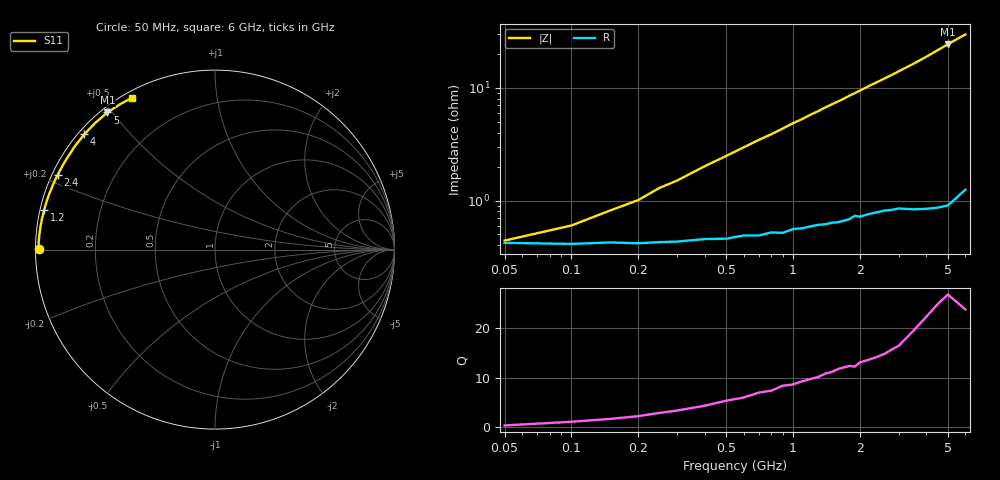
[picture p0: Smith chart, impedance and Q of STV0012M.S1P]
! SIEMENS Discrete & RF Semiconductors
! BA892
! Si PIN Diode in SCD-80
! IF = 12 mA
! S-Parameters:  September  1997
# GHz  S  MA  R  50
!  f  S11
! GHz  MAG  ANG
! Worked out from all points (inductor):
!   34 points, 50 MHz to 6 GHz, reference 50 ohm
!   read as one part to ground: L = 778 pH near 300 MHz
!   highest Q = 25.3 at 5 GHz (marker M1), where L = 774 pH
!   S11 on the Smith chart (normalised r, x): 50 MHz: 0.01, +0.00; 1.2 GHz: 0.01, +0.11; 2.4 GHz: 0.02, +0.22; 4 GHz: 0.02, +0.38; 5 GHz: 0.02, +0.49; 6 GHz: 0.02, +0.59
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0.05  0.9833 179.7
0.1  0.9837 179.0
0.15  0.9832 178.4
0.2  0.9834 177.9
0.25  0.9831 177.2
0.3  0.9829 176.7
0.4  0.982 175.5
0.7  0.9807 172.2
0.8  0.9795 171.2
0.9  0.9797 170.1
1.2  0.977 166.9
1.3  0.9763 165.9
1.4  0.9761 164.8
1.6  0.9752 162.8
1.8  0.9737 160.7
1.9  0.972 159.7
2  0.9726 158.7
2.2  0.9714 156.6
2.4  0.9704 154.7
2.6  0.9697 152.7
2.8  0.9695 150.8
3  0.969 148.7
3.5  0.9702 143.8
4  0.9709 138.6
4.5  0.9712 133.3
5  0.9711 128.1
5.5  0.9675 123.1
6  0.9638 118.5
